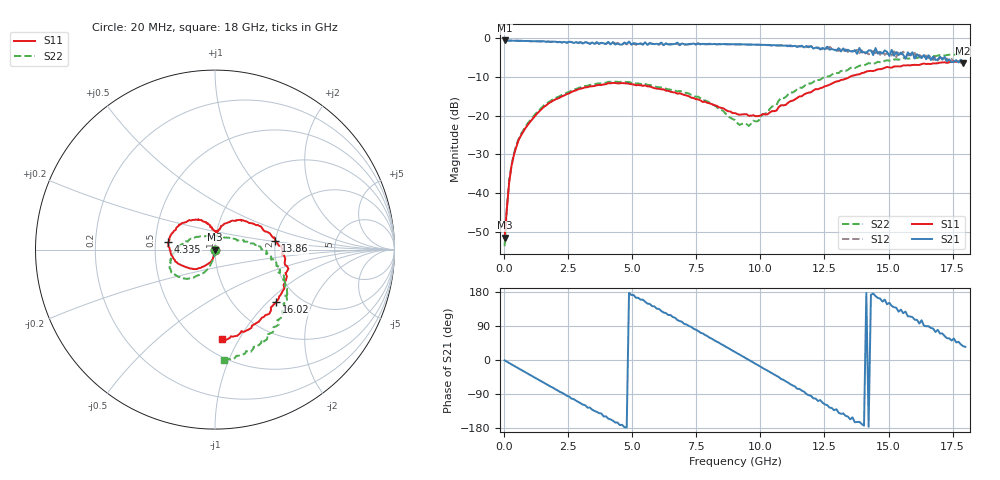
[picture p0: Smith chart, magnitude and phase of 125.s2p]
!Agilent Technologies,N5230A,US43500223,A.07.50.48
!Agilent N5230A: A.07.50.48
!Date: Saturday, January 16, 2016 21:32:22
!Correction: S11(Full 2 Port(1,2))
!S21(Full 2 Port(1,2))
!S12(Full 2 Port(1,2))
!S22(Full 2 Port(1,2))
!S2P File: Measurements: S11, S21, S12, S22:
# Hz S  dB  R 50
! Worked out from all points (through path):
!   201 points, 20 MHz to 18 GHz, reference 50 ohm
!   highest |S21| = -0.66 dB at 20 MHz (marker M1); lowest = -6.5 dB at 17.91 GHz (marker M2)
!   group delay of S21, straight-line fit = 106 ps
!   lowest |S11| = -51.5 dB at 20 MHz (marker M3), VSWR 1.01, Z = 49.7 - j0.0709 ohm
!   |S11| at or under -10 dB: start of sweep to 13.49 GHz
!   |S22| runs from -53.6 to -4.2 dB; largest |S21 - S12| = 0.15
!   S11 on the Smith chart (normalised r, x): 20 MHz: 0.99, -0.00; 4.335 GHz: 0.59, +0.05; 13.86 GHz: 2.00, +0.22; 16.02 GHz: 1.54, -1.13; 18 GHz: 0.64, -0.84
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2e7  -51.46 -164.5  -0.66 -0.9  -0.66 -0.8  -53.65 -120.3
1.998e8  -37.13 -106.3  -0.70 -8.0  -0.69 -8.1  -36.54 -97.4
6.493e8  -25.23 -103.7  -0.75 -25.4  -0.77 -25.4  -24.90 -101.3
1.9978e9  -15.86 -137.6  -0.98 -77.1  -1.01 -77.8  -15.51 -122.2
3.0766e9  -12.95 -162.1  -1.47 -117.9  -1.38 -117.3  -12.59 -136.8
4.3352e9  -11.60 171.0  -1.71 -164.9  -1.48 -164.4  -11.29 -153.5
4.8746e9  -11.80 159.9  -0.95 177.2  -1.16 177.1  -11.37 -160.8
6.0433e9  -13.10 134.3  -1.61 134.8  -1.78 135.3  -12.70 -174.5
6.7625e9  -14.37 120.2  -1.21 105.4  -1.48 105.5  -13.79 177.8
7.5716e9  -15.82 108.0  -1.45 76.8  -1.37 76.4  -15.13 165.5
9.01e9  -19.37 93.1  -1.64 21.1  -1.67 21.6  -21.17 116.4
1.03585e10  -19.25 80.2  -1.83 -31.4  -1.89 -31.0  -18.34 30.2
1.11676e10  -16.31 70.1  -1.92 -63.8  -2.15 -63.3  -14.02 9.8
1.20666e10  -13.55 51.7  -2.75 -101.1  -2.33 -98.0  -11.38 0.8
1.27858e10  -11.79 34.2  -2.86 -126.6  -2.66 -128.5  -9.47 -9.2
1.38646e10  -9.37 8.4  -2.59 -163.2  -3.93 -166.6  -7.15 -26.3
1.41343e10  -8.68 3.3  -3.89 176.8  -3.65 -175.3  -6.82 -28.5
1.50333e10  -7.61 -18.3  -4.66 151.0  -4.32 146.4  -5.86 -42.9
1.60222e10  -6.94 -40.5  -5.31 106.4  -3.84 110.5  -5.06 -57.4
1.65616e10  -6.68 -53.9  -4.46 89.1  -5.16 90.0  -4.73 -63.6
1.79101e10  -5.97 -85.2  -6.49 36.5  -6.07 38.1  -4.26 -84.1
1.8e10  -6.08 -85.7  -5.96 34.8  -6.51 36.3  -4.22 -85.4
